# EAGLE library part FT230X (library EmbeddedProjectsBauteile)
FTDI Chip USB to BASIC UART IC
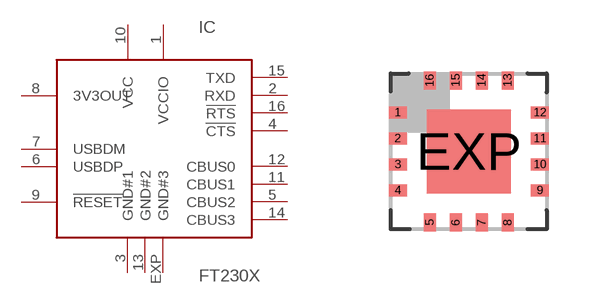
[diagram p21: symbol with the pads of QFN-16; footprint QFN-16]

Designator prefix IC

## FT230X (EP: 400870)  [QFN-16]
1  VCCIO  pwr
2  RXD
3  GND#1  pwr
4  !CTS
5  CBUS2
6  USBDP
7  USBDM
8  3V3OUT  out
9  !RESET  in
10  VCC  pwr
11  CBUS1
12  CBUS0
13  GND#2  pwr
14  CBUS3
15  TXD
16  !RTS
EXP  GND#3  pwr

## Footprint QFN-16 (pad centres in mm)
smd 0.45 x 0.3: 1 -1.78,0.975; 2 -1.78,0.325; 3 -1.78,-0.325; 4 -1.78,-0.975; 9 1.78,-0.975; 10 1.78,-0.325; 11 1.78,0.325; 12 1.78,0.975
smd 0.3 x 0.45: 5 -0.975,-1.78; 6 -0.325,-1.78; 7 0.325,-1.78; 8 0.975,-1.78; 13 0.975,1.78; 14 0.325,1.78; 15 -0.325,1.78; 16 -0.975,1.78
smd 2.1 x 2.1: EXP 0,0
